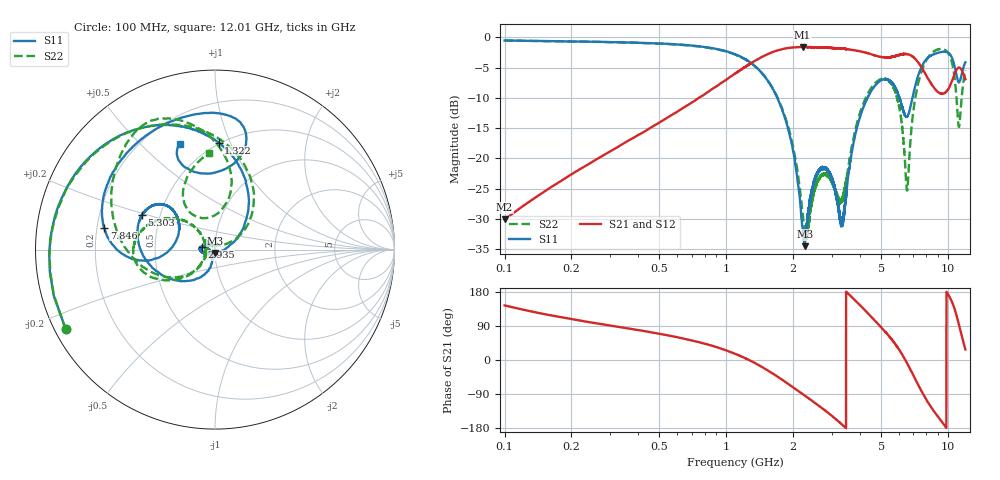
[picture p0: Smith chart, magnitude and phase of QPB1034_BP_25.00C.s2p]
! TDS: k:\Engsetup\Winsaw\QPB1034_ALL
! Channel 1
! Ports=1 2
! seg 1=100.000000 1100.000000 51
! seg 2=1101.000000 1301.000000 201
! seg 3=1302.000000 2302.000000 101
! seg 4=2303.000000 3503.000000 1201
! seg 5=3504.000000 5204.000000 171
! seg 6=5205.000000 6405.000000 1201
! seg 7=6406.000000 8506.000000 211
! seg 8=8507.000000 12007.000000 176
! Points=3313
! FailCode=0
! Topology=ALL_SE(12)
!VNA Cal loaded =QPB1034_ALL_25C
!PS1(V)= 5.000
!PS(mA)= 0.626
!PS2(V)= 1.170
!PS(mA)= -0.001
!PS3(V)= 1.170
!PS(mA)= 0.000
!PS4(V)= 1.170
!PS(mA)= -0.001
!Temp (C)= 25.00
# MHz S DB R 50
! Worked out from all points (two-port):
!   3313 points, 100 MHz to 12.01 GHz, reference 50 ohm
!   highest |S21| = -1.58 dB at 2.212 GHz (marker M1); lowest = -30.1 dB at 100 MHz (marker M2)
!   |S21| within 3 dB of the highest: 1.254 GHz to 7.499 GHz (6.245 GHz wide, 143 % of centre)
!   lowest |S11| = -34.5 dB at 2.262 GHz (marker M3), VSWR 1.04, Z = 50 - j1.88 ohm
!   |S11| at or under -10 dB: 1.702 GHz to 4.338 GHz (2.636 GHz wide, 87.3 % of centre); 6.051 GHz to 6.929 GHz (877.5 MHz wide, 13.5 % of centre)
!   |S22| runs from -33.4 to -0.5 dB; largest |S21 - S12| = 0.0066
!   S11 on the Smith chart (normalised r, x): 100 MHz: 0.03, -0.25; 1.322 GHz: 0.49, +0.91; 2.935 GHz: 0.86, +0.03; 5.303 GHz: 0.40, +0.19; 7.846 GHz: 0.23, +0.09; 12.01 GHz: 0.35, +0.67
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100  -0.51 -152.0  -30.12 144.0  -30.10 144.0  -0.51 -151.9
240  -0.71 178.9  -20.94 100.0  -20.92 100.0  -0.73 179.4
500  -1.01 154.5  -14.07 69.2  -14.07 69.1  -1.03 155.1
1100  -2.81 107.5  -5.94 16.1  -5.95 16.0  -2.85 105.4
1322  -4.48 88.1  -4.04 -5.3  -4.05 -5.7  -4.52 84.3
1802  -12.29 44.1  -1.91 -53.4  -1.91 -53.4  -12.13 39.6
2212  -31.48 -41.2  -1.58 -89.9  -1.60 -89.7  -29.14 42.9
2262  -34.53 -90.2  -1.58 -93.8  -1.59 -93.9  -32.50 66.1
2434  -25.27 -156.1  -1.63 -107.2  -1.60 -107.3  -27.56 137.7
2935  -22.38 168.3  -1.74 -143.1  -1.74 -143.1  -23.23 136.9
3328  -31.06 -156.6  -1.85 -170.1  -1.84 -170.1  -27.12 -172.3
4024  -13.10 -128.6  -2.30 144.4  -2.30 144.3  -12.34 -139.1
5303  -6.92 154.4  -3.33 70.0  -3.33 69.8  -6.95 174.6
5406  -7.04 150.4  -3.32 64.3  -3.29 64.3  -7.18 170.3
6043  -9.92 136.8  -2.89 26.6  -2.91 26.4  -11.61 139.7
6536  -13.13 163.7  -2.78 -7.3  -2.74 -7.4  -25.27 172.9
7156  -7.77 -171.4  -3.59 -52.0  -3.62 -52.0  -9.70 -153.0
7846  -4.01 168.8  -5.78 -96.2  -5.76 -96.4  -4.41 161.3
9287  -2.44 107.1  -9.32 -159.1  -9.28 -159.1  -1.91 118.7
10507  -3.61 74.7  -6.98 149.6  -6.97 150.0  -4.58 89.3
11227  -7.41 94.2  -4.99 92.9  -4.95 93.1  -14.79 101.4
12007  -4.12 108.3  -6.92 27.7  -6.93 27.9  -5.40 93.6
